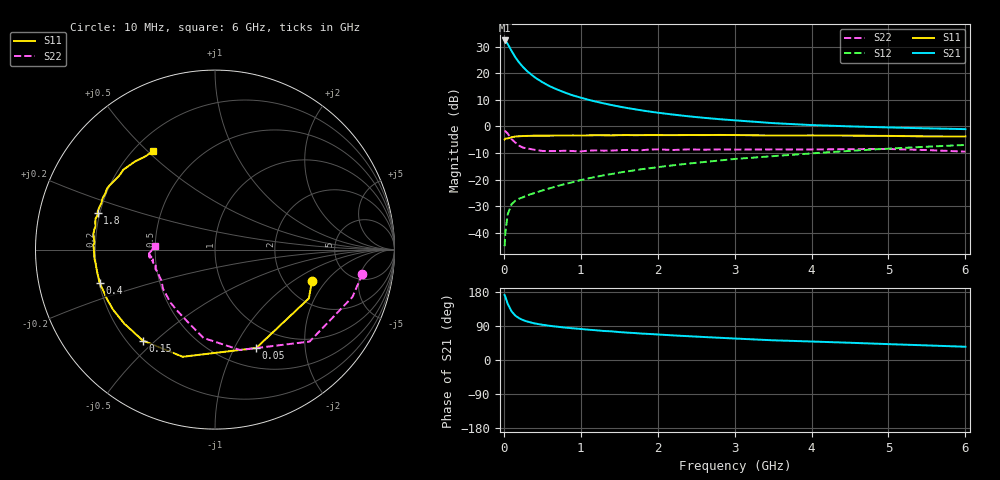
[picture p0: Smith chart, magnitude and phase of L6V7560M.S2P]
!  INFINEON TECHNOLOGIES Small Signal Semiconductors
! BFR380L3 , Si-NPN RF-Transistor in TSLP-3-1
!  Vce=0.75 V,  Ic=60 mA
! Common Emitter S-Parameters:  07. March 2005
#  GHz  S  MA  R  50
! f  S11  S21  S12  S22
! GHz  Mag  Ang  Mag  Ang  Mag  Ang  Mag  Ang
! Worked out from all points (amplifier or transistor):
!   36 points, 10 MHz to 6 GHz, reference 50 ohm
!   highest |S21| = 32.3 dB at 10 MHz (marker M1)
!   |S21| within 3 dB of that: start of sweep to 82.67 MHz
!   unconditionally stable (mu >= 1): 855.9 MHz to end of sweep
!   at 250 MHz: K = 0.56, MSG = 24.5 dB, |S12| = -26.6 dB
!   at 1.4 GHz: K = 1.08, MAG = 11.3 dB, |S12| = -17.9 dB
!   at 6 GHz: K = 1.03, MAG = 2.0 dB, |S12| = -7.0 dB
!   S11 on the Smith chart (normalised r, x): 10 MHz: 2.80, -1.45; 50 MHz: 0.72, -1.23; 150 MHz: 0.26, -0.46; 400 MHz: 0.20, -0.14; 1.8 GHz: 0.19, +0.15; 6 GHz: 0.28, +0.52
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0.01  0.5681 -17.9  41.26 171.3  0.0056 68.0  0.8323 -9.3
0.02  0.5893 -27.5  40.51 166.6  0.0102 72.4  0.8102 -19.0
0.05  0.5944 -67.3  35.45 148.3  0.0222 62.2  0.735 -44.2
0.1  0.6237 -106.8  26.36 128.6  0.0343 48.5  0.5766 -76.0
0.15  0.6469 -128.4  19.92 117.0  0.0401 43.9  0.4965 -97.4
0.2  0.6523 -140.7  15.78 110.1  0.0439 43.4  0.4321 -110.3
0.25  0.6591 -149.4  13.04 105.2  0.0466 42.7  0.3982 -122.9
0.3  0.6616 -155.0  11 101.7  0.0503 44.1  0.3857 -130.0
0.4  0.6686 -163.7  8.403 96.5  0.056 46.9  0.3629 -142.9
0.5  0.6685 -169.2  6.792 93.0  0.0624 50.3  0.3455 -149.5
0.6  0.6694 -173.1  5.652 90.1  0.0688 52.6  0.3436 -154.2
0.7  0.6736 -175.8  4.888 87.7  0.076 55.5  0.3442 -158.6
0.9  0.6773 178.0  3.814 83.6  0.0896 58.5  0.3439 -164.6
1.1  0.6789 174.4  3.162 80.0  0.1055 60.6  0.35 -166.6
1.4  0.6782 169.1  2.52 75.6  0.1272 62.1  0.3507 -169.9
1.8  0.6851 162.7  1.993 69.6  0.1572 62.8  0.3576 -173.1
2.2  0.684 157.7  1.668 64.9  0.1855 62.8  0.3601 -173.7
2.8  0.6908 150.3  1.368 58.7  0.228 62.5  0.3688 -176.2
3.5  0.6741 142.4  1.152 52.0  0.2758 59.9  0.3688 -175.9
4.5  0.6698 135.9  1 45.5  0.3468 57.1  0.3731 -175.8
5.5  0.6487 127.3  0.919 38.5  0.4153 52.2  0.3589 -178.1
6  0.6476 122.1  0.888 35.0  0.4481 49.5  0.3351 176.6
